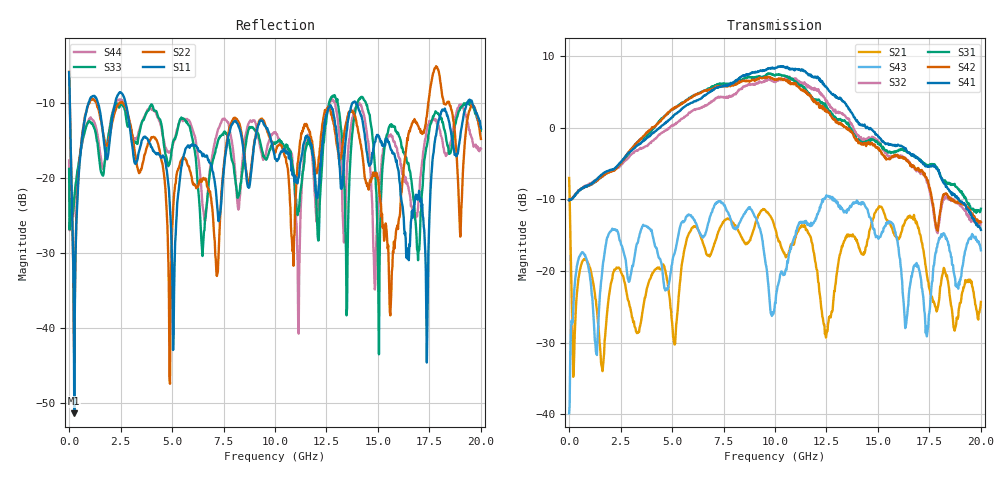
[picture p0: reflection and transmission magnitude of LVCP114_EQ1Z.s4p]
!Agilent Technologies,N5230A,MY46400459,A.07.50.48
!Agilent N5230A: A.07.50.48
!Date: Monday, January 09, 2012 14:03:00
!Correction: S11(Full 4 Port(1,2,3,4))
!S12(Full 4 Port(1,2,3,4))
!S13(Full 4 Port(1,2,3,4))
!S14(Full 4 Port(1,2,3,4))
!S21(Full 4 Port(1,2,3,4))
!S22(Full 4 Port(1,2,3,4))
!S23(Full 4 Port(1,2,3,4))
!S24(Full 4 Port(1,2,3,4))
!S31(Full 4 Port(1,2,3,4))
!S32(Full 4 Port(1,2,3,4))
!S33(Full 4 Port(1,2,3,4))
!S34(Full 4 Port(1,2,3,4))
!S41(Full 4 Port(1,2,3,4))
!S42(Full 4 Port(1,2,3,4))
!S43(Full 4 Port(1,2,3,4))
!S44(Full 4 Port(1,2,3,4))
!S4P File: Measurements: <S11,S12,S13,S14>,
!<S21,S22,S23,S24>,
!<S31,S32,S33,S34>,
!<S41,S42,S43,S44>:
# Hz S  dB  R 50
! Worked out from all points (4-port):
!   801 points, 300 kHz to 20 GHz, reference 50 ohm
!   strongest paths, dB at 300 kHz, 5 GHz, 10 GHz, 15 GHz, 20 GHz:
!     S41: -10.1, 1.5, 8.3, -1.1, -14.3
!     S42: -10.1, 2.6, 6.7, -2.9, -13.2
!     S31: -10.1, 2.6, 7.3, -2.3, -11.3
!     S32: -10.0, 0.3, 6.4, -2.0, -13.2
!     S43: -39.9, -19.1, -24.4, -15.2, -17.1
!     S21: -7.0, -27.1, -14.0, -11.3, -24.3
!   lowest |S11| = -51.4 dB at 250.3 MHz (marker M1), VSWR 1.01, Z = 50.2 + j0.107 ohm
!   |S11| at or under -10 dB: 34.51 MHz to 950 MHz (915.4 MHz wide, 186 % of centre); 2.737 GHz to 13.79 GHz (11.05 GHz wide, 134 % of centre); 13.93 GHz to 19.37 GHz (5.446 GHz wide, 32.7 % of centre)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
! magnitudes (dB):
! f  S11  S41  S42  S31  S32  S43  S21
! 300 kHz  -6.0  -10.1  -10.1  -10.1  -10.0  -39.9  -7.0
! 250.3 MHz  -51.4  -9.6  -9.5  -9.6  -9.5  -22.7  -31.0
! 1.15 GHz  -9.1  -7.7  -7.7  -7.8  -7.5  -24.7  -21.4
! 4.9 GHz  -23.9  1.2  2.3  2.3  0.1  -20.8  -24.1
! 13.88 GHz  -9.9  1.4  -1.5  -1.1  -0.6  -10.4  -15.2
! 17.38 GHz  -44.6  -5.4  -7.2  -5.3  -7.6  -29.1  -20.5
! 20 GHz  -13.4  -14.3  -13.2  -11.3  -13.2  -17.1  -24.3
